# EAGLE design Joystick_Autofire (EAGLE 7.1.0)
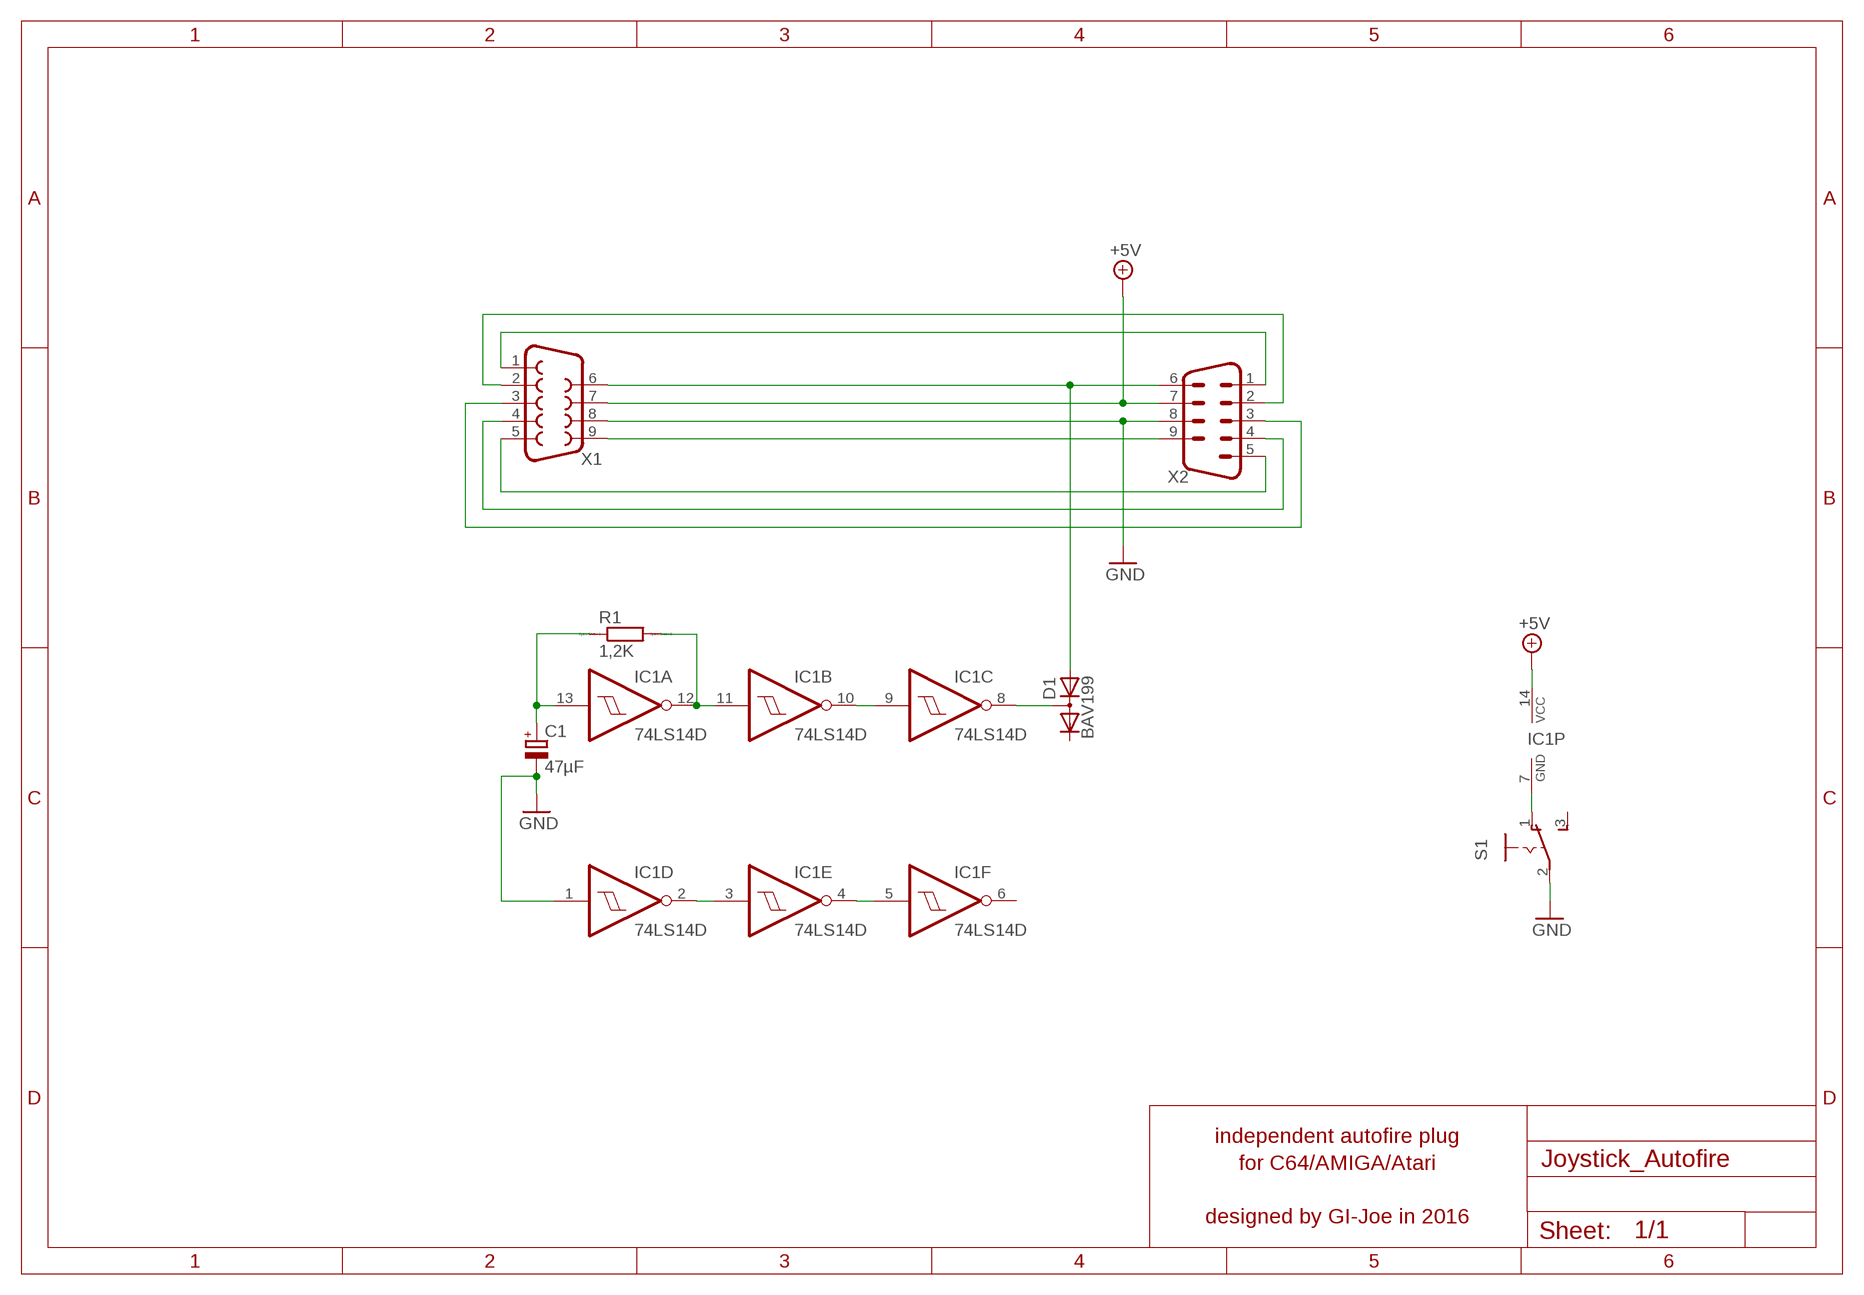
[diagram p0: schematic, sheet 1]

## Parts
C1  47µF  CPOL-EUCT3528  [CT3528]
D1  BAV199  [SOT23]
IC1  74LS14D  [SO14]
R1  1,2K  R-EU_M1206  [M1206]
S1  255SB13ASP  [255SB]
X1  F09D  [F09D]
X2  M09D  [M09D]

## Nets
+5V: IC1.14(P:VCC) X1.7 X2.7
GND: C1.- IC1.1(D:I) S1.2(P) X1.8 X2.8
N$1: D1.1(A) X1.6 X2.6
N$2: IC1.2(D:O) IC1.3(E:I)
N$3: IC1.4(E:O) IC1.5(F:I)
N$4: X1.9 X2.9
N$5: X1.5 X2.5
N$6: X1.4 X2.4
N$7: X1.3 X2.3
N$8: X1.1 X2.1
N$9: X1.2 X2.2
N$10: IC1.9(C:I) IC1.10(B:O)
N$11: D1.3(AC) IC1.8(C:O)
N$12: IC1.11(B:I) IC1.12(A:O) R1.2
N$13: IC1.7(P:GND) S1.1(O)
N$15: C1.+ IC1.13(A:I) R1.1
Unconnected: D1.2(C) IC1.6(F:O) S1.3(S)

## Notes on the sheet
- independent autofire plug
  for C64/AMIGA/Atari
  
  designed by GI-Joe in 2016

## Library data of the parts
C1 = resistor:CPOL-EU: POLARIZED CAPACITOR, European symbol
D1 = diode:BAV199: DIODE low-leakage double diode
IC1 = 74xx-eu:74*14: Hex schmitt trigger INVERTER
R1 = resistor:R-EU_: RESISTOR, European symbol; SPICEPREFIX: R
S1 = Switch_SS 13ASP:255SB: SLIDING SWITCH Distributor Reichelt, SS 13ASP
X1 = con-subd:F09: SUB-D; OC_FARNELL: unknown; OC_NEWARK: unknown
X2 = con-subd:M09: SUB-D; OC_FARNELL: unknown; OC_NEWARK: unknown

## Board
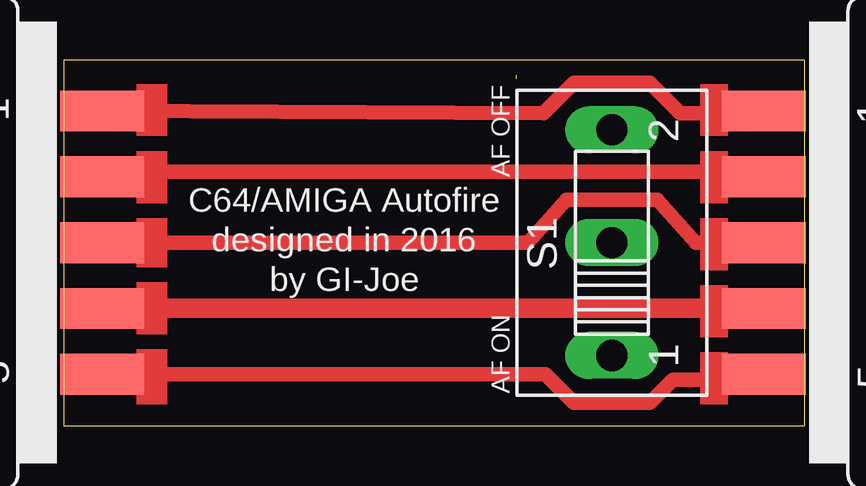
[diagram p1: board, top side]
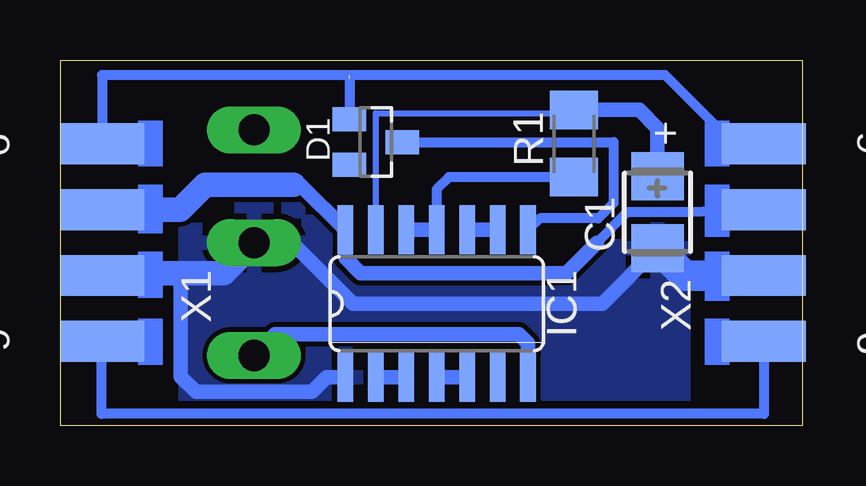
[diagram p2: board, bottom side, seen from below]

Size 30.91 x 15.23 mm. Coordinates in mm from the lower left corner, seen from the top.
Outline: 0,0 30.91,0 30.91,15.23 0,15.23 0,0
Copper layers (1*16): Top 0.035mm / dielectric 1.5mm / Bottom 0.035mm
Design rules "default": minimum track width 10mil, minimum drill 24mil, track to track 8mil, track to pad 8mil, pad to pad 8mil, via to via 8mil, smd to smd 8mil, copper to edge 40mil, drill to drill 8mil, minimum pad ring 10mil, minimum via ring 8mil, stop-mask expansion 4mil, vias tented up to drill 0mil, thermal gap 10mil

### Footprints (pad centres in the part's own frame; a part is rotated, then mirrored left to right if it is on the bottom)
CT3528 = smd 2 x 2.2: + 1.5,0; - -1.5,0
SOT23 = smd 1 x 1.4: 1 -0.95,-1.1; 2 0.95,-1.1; 3 0,1.1
SO14 = smd 0.66 x 2.032: 1 -3.81,-3.073; 2 -2.54,-3.073; 3 -1.27,-3.073; 4 0,-3.073; 5 1.27,-3.073; 6 2.54,-3.073; 7 3.81,-3.073; 8 3.81,3.073; 9 2.54,3.073; 10 1.27,3.073; 11 0,3.073; 12 -1.27,3.073; 13 -2.54,3.073; 14 -3.81,3.073
M1206 = smd 1.6 x 2: 1 -1.4,0; 2 1.4,0
255SB = drill 1.3 pad 1.7 long: 1 -4.699,0; 2 0,0; 3 4.699,0
F09D = smd 1.7 x 3.5: 1 -5.486,-6.045; 2 -2.743,-6.045; 3 0,-6.045; 4 2.743,-6.045; 5 5.486,-6.045 | smd 1.7 x 3.5 bottom: 6 -4.115,-6.045; 7 -1.372,-6.045; 8 1.372,-6.045; 9 4.115,-6.045
M09D = smd 1.7 x 3.5: 1 5.486,-6.045; 2 2.743,-6.045; 3 0,-6.045; 4 -2.743,-6.045; 5 -5.486,-6.045 | smd 1.7 x 3.5 bottom: 6 4.115,-6.045; 7 1.372,-6.045; 8 -1.372,-6.045; 9 -4.115,-6.045

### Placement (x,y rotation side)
C1  6.03,8.89 90 bottom
D1  17.78,11.81 270 bottom
IC1  15.24,5.08 0 bottom
R1  9.53,11.75 270 bottom
S1  22.86,7.62 90 top
X1  35.24,7.62 270 top
X2  -4.45,7.62 90 top

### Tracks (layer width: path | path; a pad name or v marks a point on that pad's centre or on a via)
+5V
  Bottom 0.406: X2.7 4.76,8.89 7.3,8.89 8.57,7.62
  Bottom 0.61: 8.57,7.62 9.84,6.35 18.41,6.35 19.05,6.99 IC1.14 | IC1.14 19.05,8.51 | 21.21,10.03 20.93,10.03 IC1.14
  Bottom 1.016: X1.7 25.93,8.99 24.89,10.03 21.21,10.03
GND
  Bottom 0.61: C1.- 8.34,5.08 18.73,5.08 21.27,7.62 S1.2 | 27.3,6.35 29.1,6.35 X1.8 | IC1.1 19.84,2.01 20.45,1.4 25.27,1.4 25.91,2.03 25.91,6.35
  Bottom 1.016: 27.3,6.35 25.91,6.35 24.13,6.35 S1.2
  Bottom 1.27: X2.8 4.89,6.25 C1.-
  pour Bottom: 4.95,14.61 25.72,14.61 25.72,0.64 4.95,0.64
N$1  (1 unrouted)
  Bottom 0.406: X2.6 2.85,11.73 5.71,14.61 18.73,14.61 18.88,14.46 | X1.6 29.2,14.61 18.88,14.61 D1.1
N$2
  Bottom 0.61: IC1.3 IC1.2
N$3
  Bottom 0.61: IC1.5 IC1.4
N$4
  Bottom 0.406: X2.9 1.6,0.48 29.21,0.48 X1.9
N$5
  Top 0.61: X2.5 20.09,2.13 21.27,0.95 24.45,0.95 25.4,1.91 28.97,1.91 X1.5
N$6
  Top 0.813: X1.4 X2.4
N$7
  Top 0.61: X2.3 19.37,7.62 20.95,9.4 24.77,9.4 26.35,7.62 X1.3
N$8
  Top 0.61: X2.1 20,13.02 21.27,14.29 24.45,14.29 25.72,13.02 29.11,13.02 X1.1
N$9
  Top 0.61: X2.2 1.71,10.57 29.2,10.57 X1.2
N$10
  Bottom 0.61: IC1.9 IC1.10
N$11
  Bottom 0.406: D1.3 7.87,11.81 7.87,9.27 8.51,8.64 10.95,8.64 IC1.8
N$12
  Bottom 0.406: R1.2 14.73,10.35 15.24,9.84 IC1.11
  Bottom 0.61: IC1.11 IC1.12
N$13
  Bottom 0.61: IC1.7 11.43,3.43 11.81,3.81 21.97,3.81 S1.1
N$15
  Bottom 0.254: IC1.13 17.78,13.02 9.65,13.02 R1.1
  Bottom 0.61: R1.1 6.8,13.15 6.03,12.38 C1.+
(copper drawn outside any net)
  shapes: Bottom area x8, Top area x10

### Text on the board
bPlace: +
tNames: AF OFF | C64/AMIGA Autofire | designed in 2016 | by GI-Joe | AF ON
_tNames: X1 | X1 | X2 | X2 | S1 | S1
_bNames: R1 | R1 | D1 | D1 | C1 | C1 | IC1 | IC1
